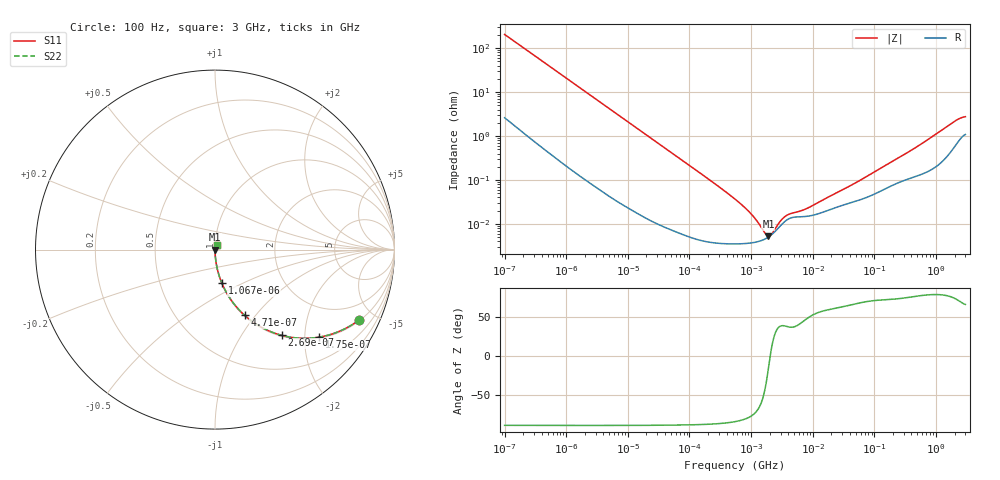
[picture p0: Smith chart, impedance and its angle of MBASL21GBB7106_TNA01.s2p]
! MBASL21GBB7106_TNA01  S-PARAMETER MODEL  ( Standard Model )
! Model Generated by TAIYO YUDEN Corporation (http://www.ty-top.com)
! Version 2.0
! TAIYO YUDEN Control No. 230906
! Copyright(c) 2020 TAIYO YUDEN CO.,LTD. All Rights Reserved.
! Product Description (link to TY-COMPAS)
! https://ds.yuden.co.jp/TYCOMPAS/or/detail?pn=MBASL21GBB7106KTNA01&u=M
! Products Name : Multilayer Ceramic Capacitors
! Characteristics :
!  Capacitance : 10 [uF] , Rated Voltage : 10 [V] , TCC : X7R
!  Case Size : 2.0 x 1.25 / 0.079 x 0.049 [mm/inch] , Thickness : 1.25 / 0.049 [mm/inch]
!  (Conditions: Temperature = 25 [degC] , DC Bias Voltage = 0 [V])
! External Node Assignments :
!  1  o---| |---o  2
! GND o---------o GND
! Frequency Range : 100Hz  -  3GHz  [ 401 STEP ]
# MHZ S RI R 50
! Freq[MHz].  S11 Real  S11 Imag  S21 Real  S21 Imag  S12 Real  S12 Imag  S22 Real  S22 Imag
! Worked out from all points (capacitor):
!   401 points, 100 Hz to 3 GHz, reference 50 ohm
!   read as one part in series: C = 7.75 uF near 109 Hz
!   lowest |Z| = 5.21 mohm at 1.908 MHz (marker M1)
!   series resonance near 2.04 MHz, so ESL is about 790 pH
!   S11 on the Smith chart (normalised r, x): 100 Hz: 1.05, -4.10; 175 Hz: 1.03, -2.35; 269 Hz: 1.02, -1.53; 471 Hz: 1.01, -0.88; 1.067 kHz: 1.00, -0.39; 3 GHz: 1.02, +0.05
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0.0001  0.8044 -0.3903  0.1956 0.3903  0.1956 0.3903  0.8044 -0.3903
0.000175  0.5794 -0.4878  0.4206 0.4878  0.4206 0.4878  0.5794 -0.4878
0.000269  0.3717 -0.4777  0.6283 0.4777  0.6283 0.4777  0.3717 -0.4777
0.000471  0.1647 -0.3657  0.8353 0.3657  0.8353 0.3657  0.1647 -0.3657
0.000664  0.0913 -0.283  0.9087 0.283  0.9087 0.283  0.0913 -0.283
0.001067  0.0384 -0.1873  0.9616 0.1873  0.9616 0.1873  0.0384 -0.1873
0.001788  0.0145 -0.1149  0.9855 0.1149  0.9855 0.1149  0.0145 -0.1149
0.005476  0.00186 -0.0383  0.9981 0.0383  0.9981 0.0383  0.00186 -0.0383
0.031977  0.00014 -0.00664  0.9999 0.00664  0.9999 0.00664  0.00014 -0.00664
0.547723  3.51e-05 -0.000366  1 0.000366  1 0.000366  3.51e-05 -0.000366
0.87939  3.61e-05 -0.000201  1 0.000201  1 0.000201  3.61e-05 -0.000201
1.352413  4.02e-05 -9.03e-05  1 9.03e-05  1 9.03e-05  4.02e-05 -9.03e-05
1.908323  5.02e-05 -1.41e-05  0.9999 1.41e-05  0.9999 1.41e-05  5.02e-05 -1.41e-05
2.69274  7.71e-05 5.56e-05  0.9999 -5.56e-05  0.9999 -5.56e-05  7.71e-05 5.56e-05
3.966702  0.000128 9.98e-05  0.9999 -9.98e-05  0.9999 -9.98e-05  0.000128 9.98e-05
6.941223  0.000146 0.000145  0.9999 -0.000145  0.9999 -0.000145  0.000146 0.000145
9.794414  0.000156 0.000206  0.9998 -0.000206  0.9998 -0.000206  0.000156 0.000206
48.15176  0.000324 0.000776  0.9997 -0.000776  0.9997 -0.000776  0.000324 0.000776
175.1444  0.000703 0.00232  0.9993 -0.00232  0.9993 -0.00232  0.000703 0.00232
513.708  0.00129 0.00579  0.9987 -0.00579  0.9987 -0.00579  0.00129 0.00579
2036.508  0.0063 0.0209  0.9937 -0.0209  0.9937 -0.0209  0.0063 0.0209
3000  0.0113 0.0248  0.9887 -0.0248  0.9887 -0.0248  0.0113 0.0248
